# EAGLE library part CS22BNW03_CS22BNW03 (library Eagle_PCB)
PCB terminal block - MPT 0,5/ 2-2,54 - 1725656 Check prices
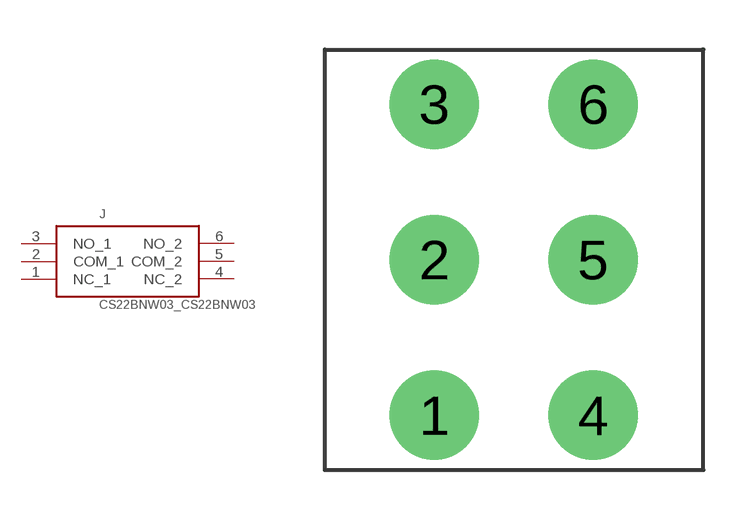
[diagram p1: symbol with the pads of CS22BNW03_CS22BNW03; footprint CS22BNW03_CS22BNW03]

Designator prefix J

## CS22BNW03_CS22BNW03 (AVAILABILITY: In Stock; DESCRIPTION: SWITCH SLIDE DPDT 3A 125V; MF: NKK Switches; MP: CS22BNW03; PACKAGE: None; PRICE: None)  [CS22BNW03_CS22BNW03]
1  NC_1
2  COM_1
3  NO_1
4  NC_2
5  COM_2
6  NO_2

## Footprint CS22BNW03_CS22BNW03 (pad centres in mm)
PCB terminal block - MPT 0,5/ 3-2,54
drill 1.8: 1 -2.4,-4.7; 2 -2.4,0; 3 -2.4,4.7; 4 2.4,-4.7; 5 2.4,0; 6 2.4,4.7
